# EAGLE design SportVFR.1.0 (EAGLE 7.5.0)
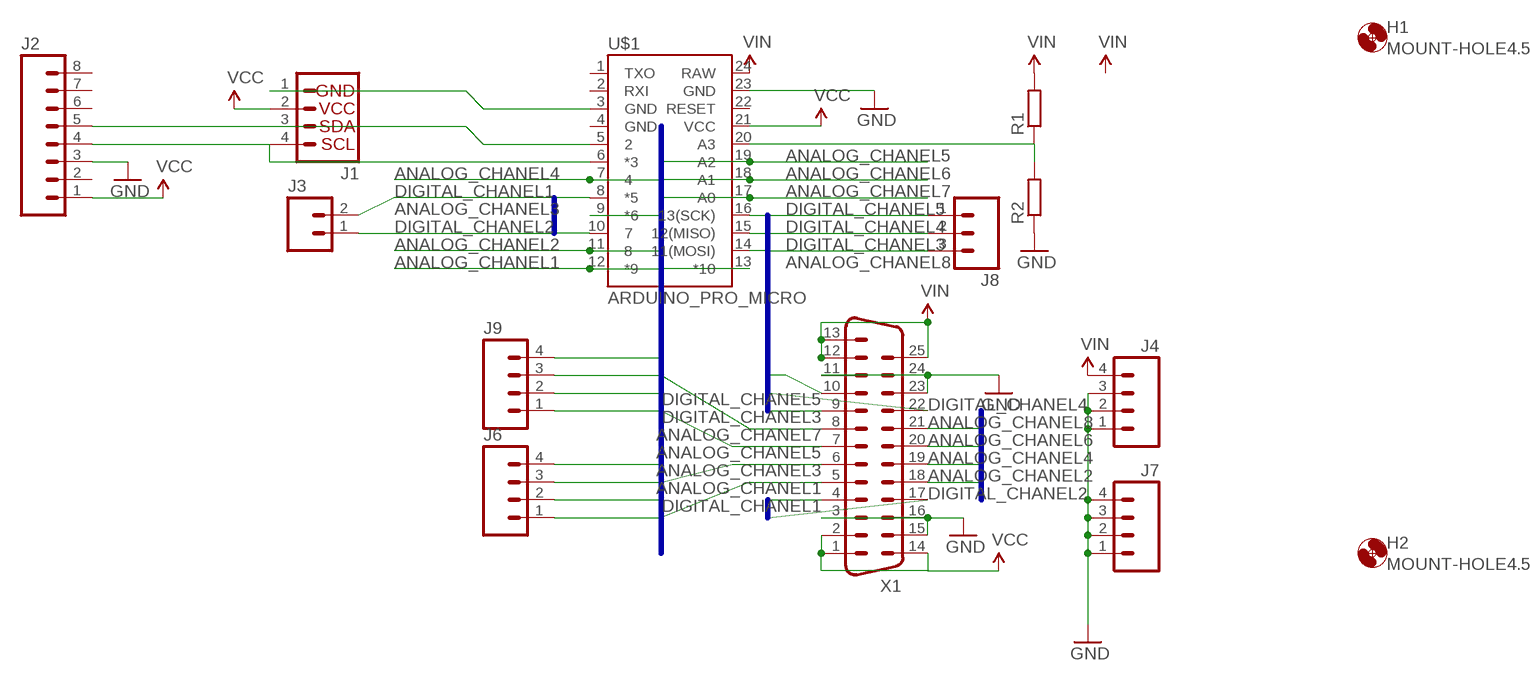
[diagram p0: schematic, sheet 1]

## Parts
H1  MOUNT-HOLE4.5  [4,5]
H2  MOUNT-HOLE4.5  [4,5]
J1  I2C_STANDARD  [1X04]
J2  M08SILK_FEMALE_PTH  [1X08]
J3  M02PTH  [1X02]
J4  M04PTH  [1X04]
J6  M04PTH  [1X04]
J7  M04PTH  [1X04]
J8  M03PTH  [1X03]
J9  M04PTH  [1X04]
R1  R-EU_R0805  [R0805]
R2  R-EU_R0805  [R0805]
U$1  ARDUINO_PRO_MICRO  [ARDUINO_PRO_MICRO]
X1  DB25HP  [M25HP]

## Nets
ANALOG_CHANEL1: J6.1 U$1.12(*9) X1.5
ANALOG_CHANEL2: J6.2 U$1.11 X1.18
ANALOG_CHANEL3: J6.3 U$1.9(*6) X1.6
ANALOG_CHANEL4: J6.4 U$1.7 X1.19
ANALOG_CHANEL5: J9.1 U$1.19(A2) X1.7
ANALOG_CHANEL6: J9.2 U$1.18(A1) X1.20
ANALOG_CHANEL7: J9.3 U$1.17(A0) X1.8
ANALOG_CHANEL8: J9.4 U$1.13(*10) X1.21
DIGITAL_CHANEL1: J3.2 U$1.8(*5) X1.4
DIGITAL_CHANEL2: J3.1 U$1.10 X1.17
DIGITAL_CHANEL3: J8.3 U$1.14(11(MOSI)) X1.9
DIGITAL_CHANEL4: J8.2 U$1.15(12(MISO)) X1.22
DIGITAL_CHANEL5: J8.1 U$1.16(13(SCK)) X1.10
GND: J2.3 J4.1 J4.2 J4.3 J7.1 J7.2 J7.3 J7.4 R2.1 U$1.23(GND) X1.3 X1.11 X1.15 X1.16 X1.23 X1.24
N$1: J1.3 J2.5 U$1.5
N$2: J1.4 J2.4 U$1.6(*3)
N$3: J1.1 U$1.3(GND)
N$9: R1.1 R2.2 U$1.20(A3)
VCC: J1.2 J2.1 U$1.21(VCC) X1.1 X1.2 X1.14
VIN: J4.4 R1.2 U$1.24(RAW) X1.12 X1.13 X1.25
Unconnected: J2.2 J2.6 J2.7 J2.8 U$1.1(TXO) U$1.2(RXI) U$1.4(GND) U$1.22(RESET)

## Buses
ANALOG_CHANEL[1..9]
DIGITAL_CHANEL[1..5]
ANALOG_CHANEL[1..8]

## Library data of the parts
H1 H2 = holes:MOUNT-HOLE: MOUNTING HOLE with drill center marker
J1 = SparkFun-Connectors:I2C_STANDARD: SparkFun has standardized on a pinout for all I2C based sensor breakouts. This pinout allows I2C boards to be plugged directly into the headers on Arduino Uno compatible boards, and to be daisy chained easily.
J2 = SparkFun-Connectors:M08: Header 8 Standard 8-pin 0.1" header. Use with straight break away headers (SKU : PRT-00116), right angle break away headers (PRT-00553), swiss pins (PRT-00743), machine pins (PRT-00117), and female headers (PRT-00115).; PROD_ID: CONN-08438
J3 = SparkFun-Connectors:M02: Standard 2-pin 0.1" header. Use with
J4 J6 J7 J9 = SparkFun-Connectors:M04: Header 4 Standard 4-pin 0.1" header. Use with straight break away headers (SKU : PRT-00116), right angle break away headers (PRT-00553), swiss pins (PRT-00743), machine pins (PRT-00117), and female headers (PRT-00115). Molex polarized connector foot print use with SKU : PRT-08231 with associated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; PROD_ID: CONN-09696
J8 = SparkFun-Connectors:M03: Header 3 Standard 3-pin 0.1" header. Use with straight break away headers (SKU : PRT-00116), right angle break away headers (PRT-00553), swiss pins (PRT-00743), machine pins (PRT-00117), and female headers (PRT-00115). Molex polarized connector foot print use with SKU : PRT-08232 with associated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
R1 R2 = resistor:R-EU_: RESISTOR, European symbol
U$1 = SparkFun-Boards:ARDUINO_PRO_MICRO
X1 = SparkFun-Connectors:DB25: Various DB25 connectors

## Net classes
0 default: clearance 0.406 mm

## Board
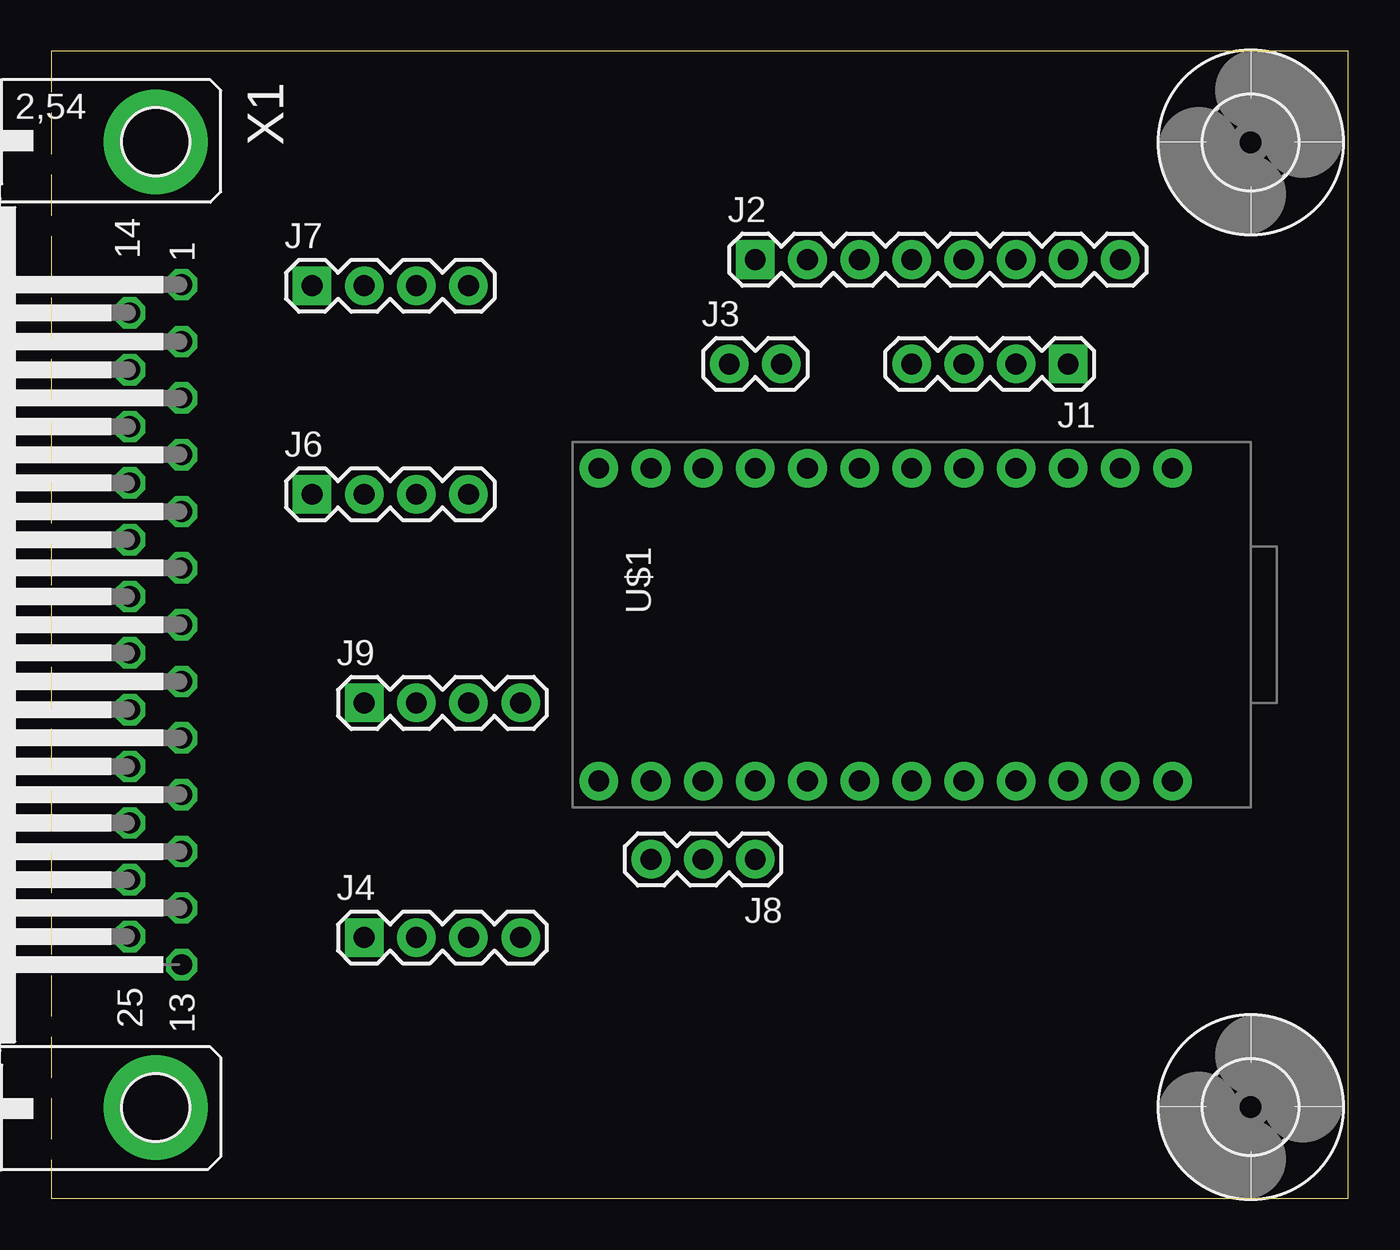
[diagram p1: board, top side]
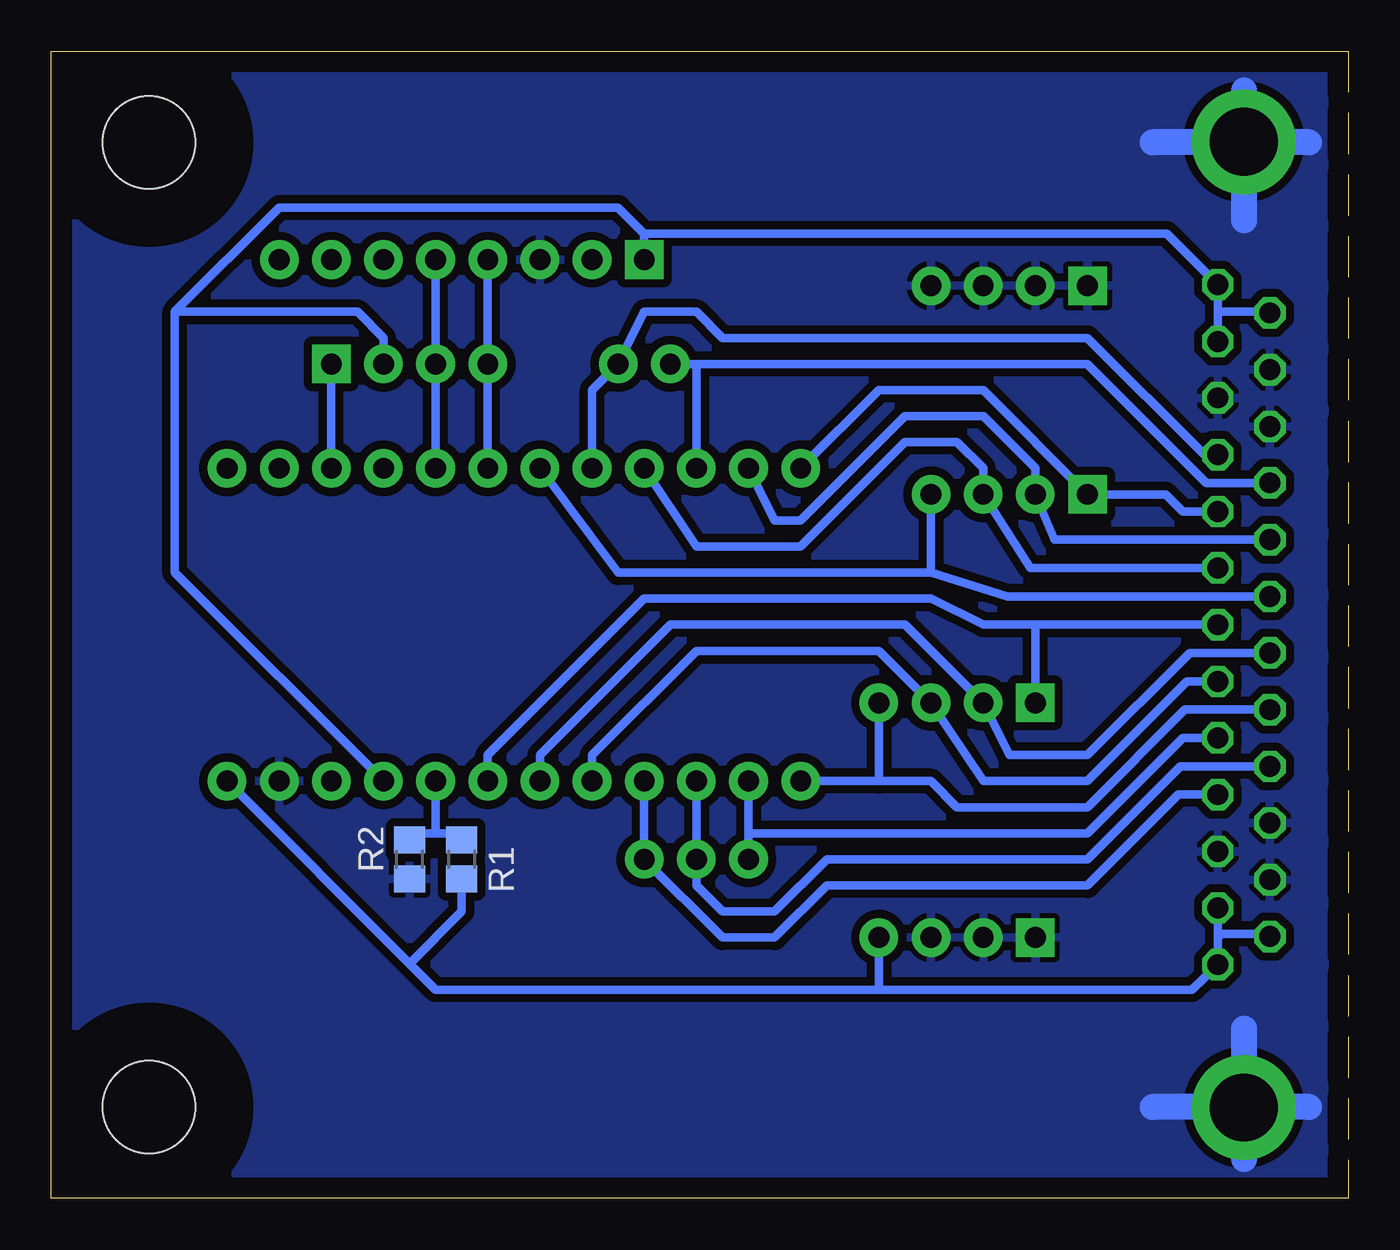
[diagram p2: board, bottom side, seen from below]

Size 63.17 x 55.87 mm. Coordinates in mm from the lower left corner, seen from the top.
Outline: 0,0 63.17,0 63.17,55.87 0,55.87 0,0
Copper layers (1*16): Top 0.035mm / dielectric 1.5mm / Bottom 0.035mm
Design rules "default": minimum track width 10mil, minimum drill 24mil, track to track 8mil, track to pad 8mil, pad to pad 8mil, via to via 8mil, smd to smd 8mil, copper to edge 40mil, drill to drill 8mil, minimum pad ring 10mil, minimum via ring 8mil, stop-mask expansion 4mil, vias tented up to drill 0mil, thermal gap 10mil

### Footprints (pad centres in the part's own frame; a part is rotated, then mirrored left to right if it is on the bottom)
4,5 = hole 4.5: 0,0
1X04 = drill 1.016 pad 1.88 square: 1 0,0 | drill 1.016 pad 1.88: 2 2.54,0; 3 5.08,0; 4 7.62,0
1X08 = drill 1.016 pad 1.88 square: 1 0,0 | drill 1.016 pad 1.88: 2 2.54,0; 3 5.08,0; 4 7.62,0; 5 10.16,0; 6 12.7,0; 7 15.24,0; 8 17.78,0
1X02 = drill 1.016 pad 1.88: 1 0,0; 2 2.54,0
1X03 = drill 1.016 pad 1.88: 1 0,0; 2 2.54,0; 3 5.08,0
R0805 = smd 1.3 x 1.5: 1 -0.95,0; 2 0.95,0
ARDUINO_PRO_MICRO = drill 1.016 pad 1.88: 1 -7.62,12.7; 2 -7.62,10.16; 3 -7.62,7.62; 4 -7.62,5.08; 5 -7.62,2.54; 6 -7.62,0; 7 -7.62,-2.54; 8 -7.62,-5.08; 9 -7.62,-7.62; 10 -7.62,-10.16; 11 -7.62,-12.7; 12 -7.62,-15.24; 13 7.62,-15.24; 14 7.62,-12.7; 15 7.62,-10.16; 16 7.62,-7.62; 17 7.62,-5.08; 18 7.62,-2.54; 19 7.62,0; 20 7.62,2.54; 21 7.62,5.08; 22 7.62,7.62; 23 7.62,10.16; 24 7.62,12.7
M25HP = drill 1.016 octagon: 1 -16.561,1.27; 2 -13.792,1.27; 3 -11.049,1.27; 4 -8.28,1.27; 5 -5.512,1.27; 6 -2.769,1.27; 7 0,1.27; 8 2.769,1.27; 9 5.512,1.27; 10 8.28,1.27; 11 11.049,1.27; 12 13.792,1.27; 13 16.561,1.27; 14 -15.189,-1.27; 15 -12.421,-1.27; 16 -9.652,-1.27; 17 -6.909,-1.27; 18 -4.14,-1.27; 19 -1.372,-1.27; 20 1.372,-1.27; 21 4.14,-1.27; 22 6.909,-1.27; 23 9.652,-1.27; 24 12.421,-1.27; 25 15.189,-1.27 | drill 3.302 pad 5.08: G1 -23.52,0; G2 23.52,0

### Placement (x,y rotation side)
H1  58.42,51.44 0 top
H2  58.42,4.45 0 top
J1  49.53,40.64 180 top
J2  34.29,45.72 0 top
J3  33.02,40.64 0 top
J4  15.24,12.7 0 top
J6  12.7,34.29 0 top
J7  12.7,44.45 0 top
J8  34.29,16.51 180 top
J9  15.24,24.13 0 top
R1  43.18,16.51 270 bottom
R2  45.72,16.51 90 bottom
U$1  41.91,27.94 270 top
X1  5.08,27.94 270 top

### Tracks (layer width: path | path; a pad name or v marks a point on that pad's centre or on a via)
ANALOG_CHANEL1
  Bottom 0.406: X1.5 8.05,33.45 8.89,34.29 J6.1 17.78,39.37 22.86,39.37 U$1.12
ANALOG_CHANEL2
  Bottom 0.406: X1.18 14.3,32.08 J6.2 15.24,35.56 17.78,38.1 21.59,38.1 26.67,33.02 27.94,33.02 U$1.11
ANALOG_CHANEL3
  Bottom 0.406: X1.6 15.47,30.71 J6.3 17.78,35.56 19.05,36.83 21.59,36.83 26.67,31.75 31.75,31.75 U$1.9
ANALOG_CHANEL4
  Bottom 0.406: 20.32,30.48 35.56,30.48 U$1.7 | X1.19 16.61,29.31 20.32,30.48 | J6.4 20.32,30.48
ANALOG_CHANEL5
  Bottom 0.406: U$1.19 41.91,21.59 34.29,29.21 20.32,29.21 17.78,27.94 15.24,27.94 | 15.24,27.94 X1.7 | J9.1 15.24,27.94
ANALOG_CHANEL6
  Bottom 0.406: X1.20 7.72,26.57 12.7,21.59 16.51,21.59 J9.2 21.59,27.94 33.02,27.94 39.37,21.59 U$1.18
ANALOG_CHANEL7
  Bottom 0.406: X1.8 7.85,25.17 12.7,20.32 17.78,20.32 J9.3 22.86,26.67 31.75,26.67 36.83,21.59 U$1.17
ANALOG_CHANEL8
  Bottom 0.406: X1.21 7.95,23.8 12.7,19.05 19.05,19.05 20.32,20.32 22.86,20.32 | 22.86,20.32 U$1.13 | J9.4 22.86,20.32
DIGITAL_CHANEL1
  Bottom 0.406: U$1.8 36.83,39.37 J3.2 34.29,43.18 31.75,43.18 30.48,41.91 12.7,41.91 7.01,36.22 X1.4
DIGITAL_CHANEL2
  Bottom 0.406: 31.75,40.64 12.7,40.64 6.91,34.85 X1.17 | J3.1 31.75,40.64 | 31.75,40.64 U$1.10
DIGITAL_CHANEL3
  Bottom 0.406: X1.9 8.05,22.43 12.7,17.78 29.21,17.78 | U$1.14 29.21,17.78 | 29.21,17.78 J8.3
DIGITAL_CHANEL4
  Bottom 0.406: U$1.15 J8.2 31.75,15.24 30.48,13.97 27.94,13.97 25.4,16.51 12.7,16.51 8.18,21.03 X1.22
DIGITAL_CHANEL5
  Bottom 0.406: U$1.16 J8.1 30.48,12.7 27.94,12.7 25.4,15.24 12.7,15.24 8.28,19.66 X1.10
GND
  Bottom 1.27: 1.91,4.45 9.53,4.45 | 5.08,8.26 5.08,1.91 | 5.08,53.98 5.08,47.62 | 1.91,51.44 9.53,51.44
  pour Bottom: 0,0 0,55.88 63.5,55.88 63.5,0
N$1
  Bottom 0.406: U$1.5 J1.3 J2.5
N$2
  Bottom 0.406: U$1.6 J1.4 J2.4
N$3
  Bottom 0.406: U$1.3 J1.1
N$9
  Bottom 0.406: U$1.20 44.45,17.78 | 44.45,17.78 43.5,17.78 R1.1 | R2.2 45.4,17.78 44.45,17.78
VCC
  Bottom 0.406: U$1.21 57.15,30.48 57.15,43.18 | 57.15,43.18 48.26,43.18 46.99,41.91 J1.2 | X1.14 3.81,43.18 6.35,43.18 | X1.2 6.35,43.18 | 6.35,43.18 X1.1 8.84,46.99 34.29,46.99 | J2.1 34.29,46.99 | 34.29,46.99 35.56,48.26 52.07,48.26 57.15,43.18
VIN
  Bottom 0.406: 22.86,10.16 7.62,10.16 X1.13 6.35,12.7 | 22.86,10.16 44.45,10.16 45.72,11.43 | 45.72,11.43 U$1.24 | X1.12 6.35,12.7 | X1.25 3.81,12.88 6.17,12.88 6.35,12.7 | R1.2 43.18,13.97 45.72,11.43 | J4.4 22.86,10.16

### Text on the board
bDocu: Innertia/Position Sensors | D1 | IIC - Display | ANALOG CH / 4 3 2 1 | 8 7 6 5 / ANALOG CH | D5 | v1.0 | SportVFR | (c) Bruce Meacham 2016

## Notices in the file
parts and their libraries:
SparkFun-Boards: Licensing: Creative Commons ShareAlike 4.0 International - https://creativecommons.org/licenses/by-sa/4.0
